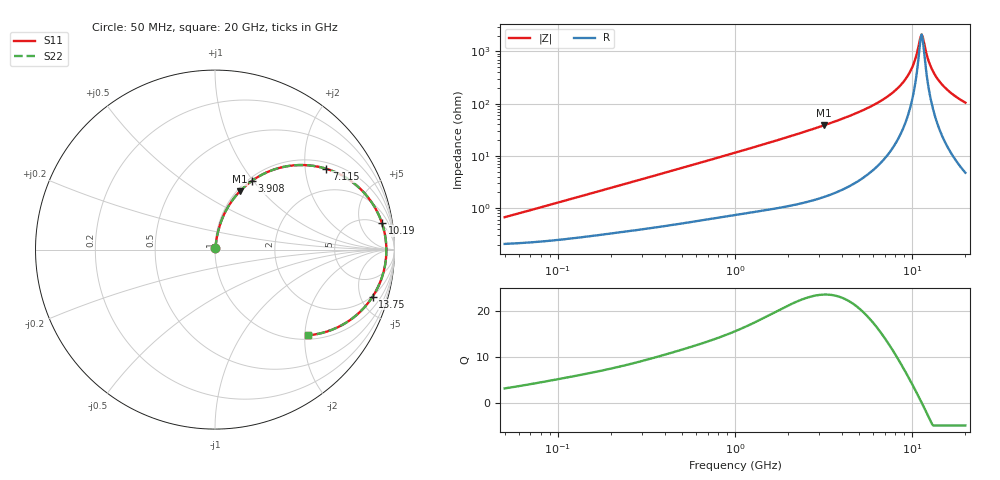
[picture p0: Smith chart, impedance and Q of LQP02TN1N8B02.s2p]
!Murata Part Number: LQP02TN1N8B02
!These Parameters are Measured in Series Mode Connection
!  o--[Z]--o
!Port1  Port2
!  o-------o
!Freq. Start=50[MHz] Stop=20[GHz], 401[Steps]
# Hz S RI R 50
!Freq.(Hz) S11(Real) S11(Imag) S21(Real) S21(Imag) S12(Real) S12(Imag) S22(Real) S22(Imag)
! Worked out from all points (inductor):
!   401 points, 50 MHz to 20 GHz, reference 50 ohm
!   read as one part in series: L = 2.01 nH near 51.52 MHz
!   highest Q = 23.6 at 3.169 GHz (marker M1), where L = 1.92 nH
!   self-resonance near 11.32 GHz
!   S11 on the Smith chart (normalised r, x): 50 MHz: 1.00, +0.01; 3.908 GHz: 1.04, +0.99; 7.115 GHz: 1.19, +2.60; 10.19 GHz: 4, +11; 13.75 GHz: 1.92, -6.27; 20 GHz: 1.09, -2.09
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5e7  0.00209 0.00633  0.9979 -0.00633  0.9979 -0.00633  0.00209 0.00633
1.364002e8  0.00304 0.0167  0.997 -0.0167  0.997 -0.0167  0.00304 0.0167
3.721004e8  0.00623 0.0434  0.9938 -0.0434  0.9938 -0.0434  0.00623 0.0434
1e9  0.02 0.1115  0.98 -0.1115  0.98 -0.1115  0.02 0.1115
2.728004e9  0.1043 0.2849  0.8957 -0.2849  0.8957 -0.2849  0.1043 0.2849
3.168813e9  0.138 0.3243  0.862 -0.3243  0.862 -0.3243  0.138 0.3243
3.908127e9  0.2057 0.3831  0.7943 -0.3831  0.7943 -0.3831  0.2057 0.3831
5.273168e9  0.3648 0.4568  0.6352 -0.4568  0.6352 -0.4568  0.3648 0.4568
7.114996e9  0.6205 0.4501  0.3795 -0.4501  0.3795 -0.4501  0.6205 0.4501
7.442007e9  0.6655 0.4337  0.3345 -0.4337  0.3345 -0.4337  0.6655 0.4337
9.041845e9  0.8515 0.2924  0.1485 -0.2924  0.1485 -0.2924  0.8515 0.2924
9.600142e9  0.8963 0.2251  0.1037 -0.2251  0.1037 -0.2251  0.8963 0.2251
1.019291e10  0.9299 0.1484  0.0701 -0.1484  0.0701 -0.1484  0.9299 0.1484
1.050288e10  0.9418 0.1073  0.0582 -0.1073  0.0582 -0.1073  0.9418 0.1073
1.098561e10  0.9525 0.0434  0.0475 -0.0434  0.0475 -0.0434  0.9525 0.0434
1.131968e10  0.9548 2.19e-05  0.0452 -2.19e-05  0.0452 -2.19e-05  0.9548 2.19e-05
1.166392e10  0.9531 -0.0434  0.0469 0.0434  0.0469 0.0434  0.9531 -0.0434
1.220001e10  0.9433 -0.1076  0.0567 0.1076  0.0567 0.1076  0.9433 -0.1076
1.257102e10  0.932 -0.149  0.068 0.149  0.068 0.149  0.932 -0.149
1.375312e10  0.8782 -0.2622  0.1218 0.2622  0.1218 0.2622  0.8782 -0.2622
1.621653e10  0.7288 -0.4082  0.2712 0.4082  0.2712 0.4082  0.7288 -0.4082
2e10  0.5208 -0.4774  0.4792 0.4774  0.4792 0.4774  0.5208 -0.4774
